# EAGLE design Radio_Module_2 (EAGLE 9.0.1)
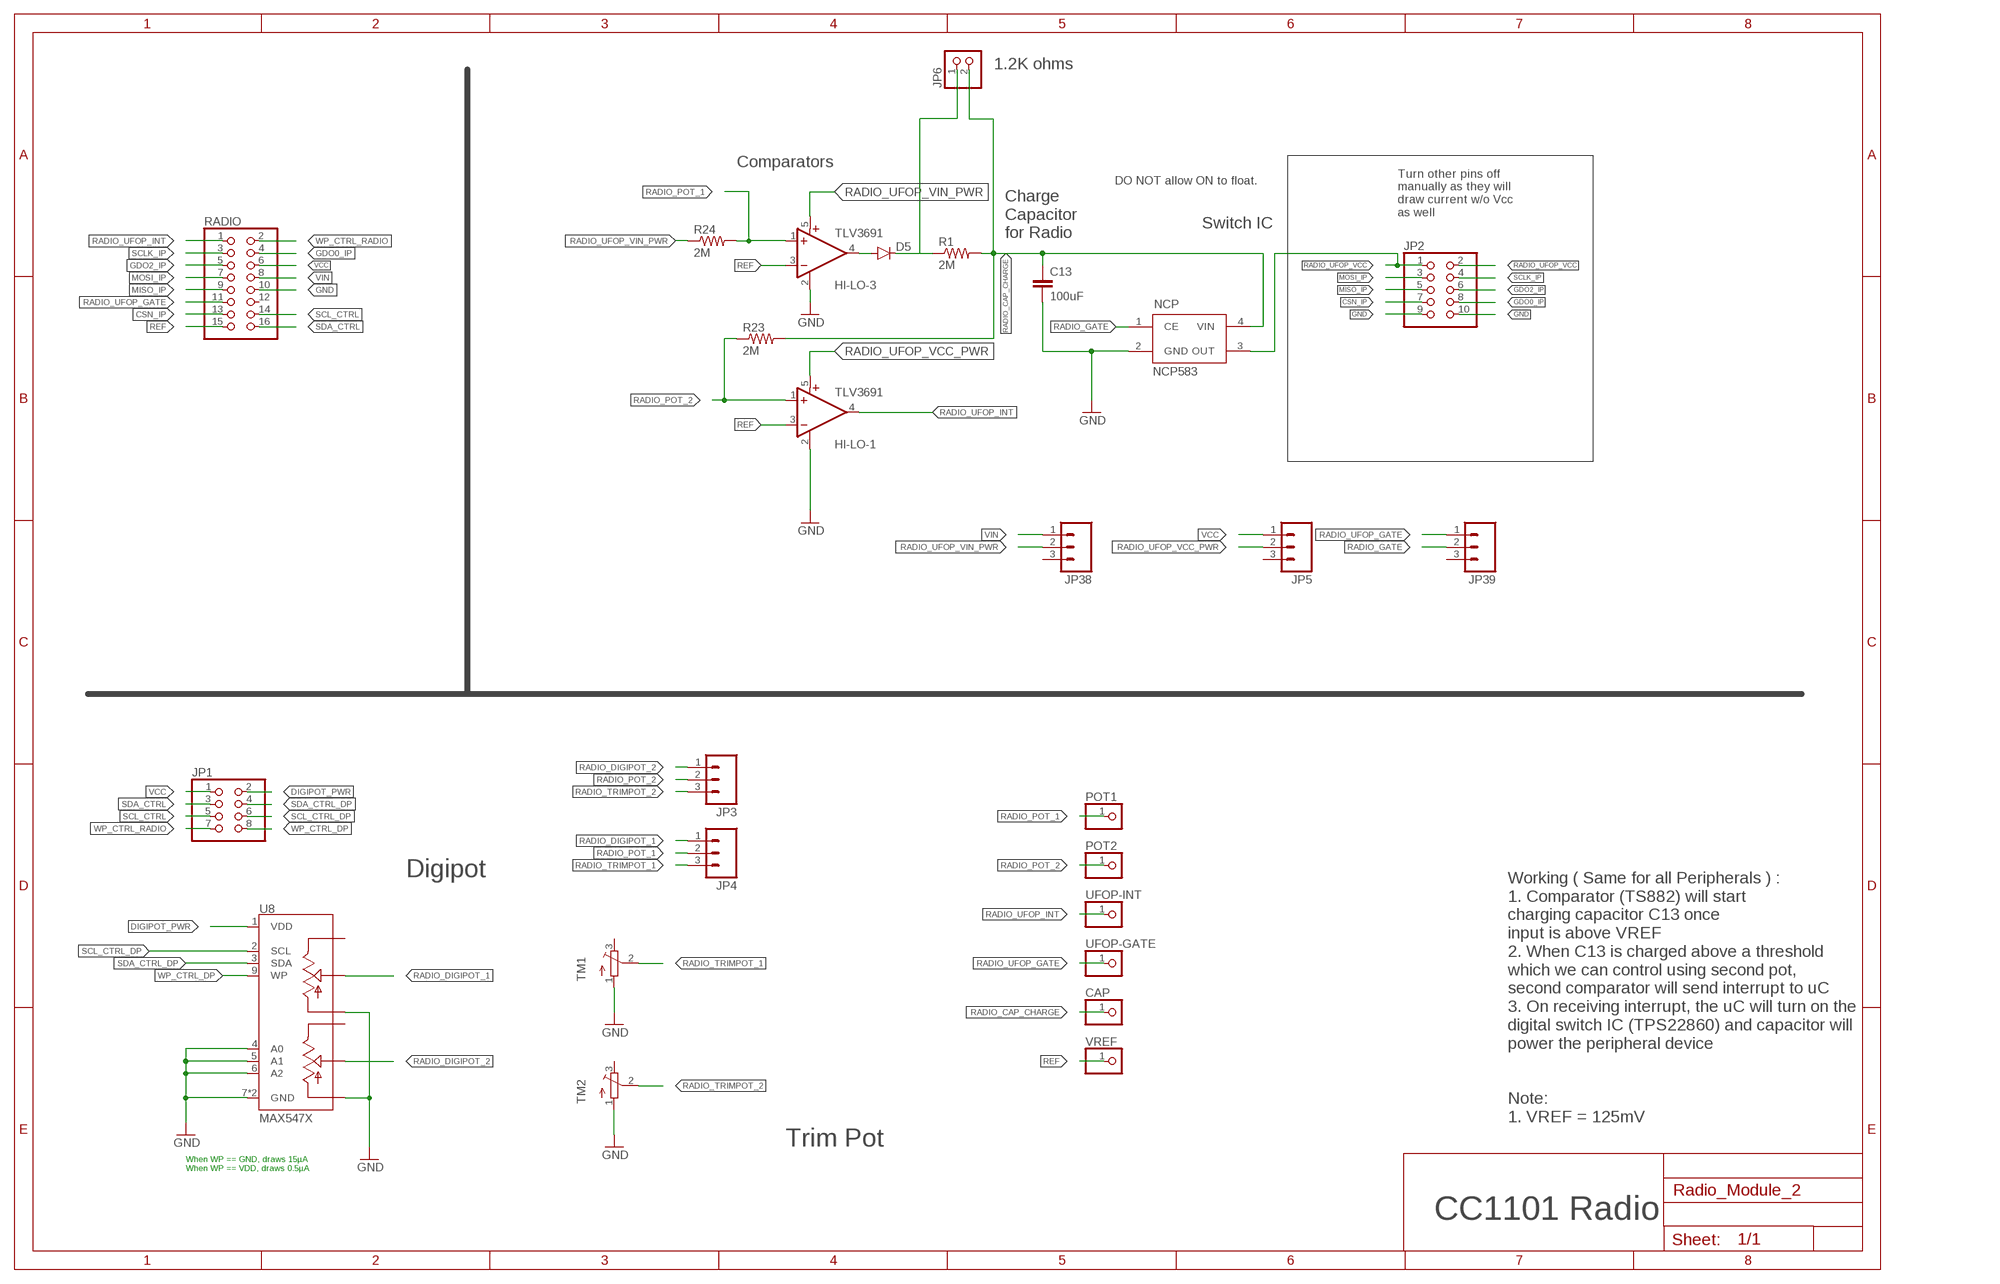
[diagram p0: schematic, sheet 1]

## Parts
C13  100uF  CAP0805  [0805]
CAP  PINHD-1X1  [1X01]
D5  DIODESOD523  [SOD523]
HI-LO-1  TLV3691  [SC70-5]
HI-LO-3  TLV3691  [SC70-5]
JP1  PINHD-2X4  [2X04]
JP2  PINHD-2X5  [2X05]
JP3  M03  [1X03-1.27MM]
JP4  M03  [1X03-1.27MM]
JP5  M03  [1X03-1.27MM]
JP6  PINHD-1X2  [1X02]
JP38  M03  [1X03-1.27MM]
JP39  M03  [1X03-1.27MM]
NCP  NCP583  [SC82-AB_1PRIMARY]
POT1  PINHD-1X1  [1X01]
POT2  PINHD-1X1  [1X01]
R1  2M  RESISTOR0805-RES  [0805]
R23  2M  RESISTOR0805-RES  [0805]
R24  2M  RESISTOR0805-RES  [0805]
RADIO  PINHD-2X8/90  [2X08/90]
TM1  TRIMPOTTC33X  [TC33X]
TM2  TRIMPOTTC33X  [TC33X]
U8  MAX547X  [QFN16]
UFOP-GATE  PINHD-1X1  [1X01]
UFOP-INT  PINHD-1X1  [1X01]
VREF  PINHD-1X1  [1X01]

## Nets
CSN_IP: JP2.7 RADIO.13
DIGIPOT_PWR: JP1.2 U8.1(VDD)
GDO0_IP: JP2.8 RADIO.4
GDO2_IP: JP2.6 RADIO.5
GND: C13.2 HI-LO-1.2(GND) HI-LO-3.2(GND) JP2.9 JP2.10 NCP.2(GND) RADIO.10 TM1.1(A) TM2.1(A) U8.4(A0) U8.5(A1) U8.6(A2) U8.7(GND) U8.10(LB) U8.13(LA) U8.TH(GND)
MISO_IP: JP2.5 RADIO.9
MOSI_IP: JP2.3 RADIO.7
N$1: D5.C JP6.1 R1.1
N$24: D5.A HI-LO-3.4(OUT)
RADIO_CAP_CHARGE: C13.1 CAP.1 JP6.2 NCP.4(VIN) R1.2 R23.2
RADIO_DIGIPOT_1: JP4.1 U8.14(WA)
RADIO_DIGIPOT_2: JP3.1 U8.11(WB)
RADIO_GATE: JP39.2 NCP.1(CE)
RADIO_POT_1: HI-LO-3.1(+IN) JP4.2 POT1.1 R24.2
RADIO_POT_2: HI-LO-1.1(+IN) JP3.2 POT2.1 R23.1
RADIO_TRIMPOT_1: JP4.3 TM1.2(S)
RADIO_TRIMPOT_2: JP3.3 TM2.2(S)
RADIO_UFOP_GATE: JP39.1 RADIO.11 UFOP-GATE.1
RADIO_UFOP_INT: HI-LO-1.4(OUT) RADIO.1 UFOP-INT.1
RADIO_UFOP_VCC: JP2.1 JP2.2 NCP.3(OUT)
RADIO_UFOP_VCC_PWR: HI-LO-1.5(V+) JP5.2
RADIO_UFOP_VIN_PWR: HI-LO-3.5(V+) JP38.2 R24.1
REF: HI-LO-1.3(-IN) HI-LO-3.3(-IN) RADIO.15 VREF.1
SCL_CTRL: JP1.5 RADIO.14
SCL_CTRL_DP: JP1.6 U8.2(SCL)
SCLK_IP: JP2.4 RADIO.3
SDA_CTRL: JP1.3 RADIO.16
SDA_CTRL_DP: JP1.4 U8.3(SDA)
VCC: JP1.1 JP5.1 RADIO.6
VIN: JP38.1 RADIO.8
WP_CTRL_DP: JP1.8 U8.9(WP)
WP_CTRL_RADIO: JP1.7 RADIO.2
Unconnected: JP5.3 JP38.3 JP39.3 RADIO.12 TM1.3(E) TM2.3(E) U8.12(HB) U8.15(HA)

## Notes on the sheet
- 1.2K ohms
- Comparators
- DO NOT allow ON to float.
- Charge 
  Capacitor 
  for Radio
- Turn other pins off 
  manually as they will
  draw current w/o Vcc
  as well
- Switch IC
- Digipot
- Working ( Same for all Peripherals ) :
  1. Comparator (TS882) will start 
  charging capacitor C13 once 
  input is above VREF
  2. When C13 is charged above a threshold
  which we can control using second pot, 
  second comparator will send interrupt to uC
  3. On receiving interrupt, the uC will turn on the
  digital switch IC (TPS22860) and capacitor will 
  power the peripheral device
- Note:
  1. VREF = 125mV
- Trim Pot
- When WP == GND, draws 15µA
  When WP == VDD, draws 0.5µA
- CC1101 Radio

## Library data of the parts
C13 = SparkFun-Capacitors:CAP: Capacitor; DIGIKEY: 490-9969-1-ND
CAP POT1 POT2 UFOP-GATE UFOP-INT VREF = adafruit:PINHD-1X1: Pin header 1x1 for 0.1" spacing
D5 = SparkFun-DiscreteSemi:DIODE: Diode
HI-LO-1 HI-LO-3 = fedpower:TLV3691: 0.9-V to 6.5-V, Nanopower Comparator Datasheets Analog Signal Chain Guide TLV3691 Manufacturer Product Page TLV3691IDPFR Specifications Standard Package 1 CategoryIntegrated Circuits (ICs) FamilyLinear - Comparators Series- Packaging Cut Tape (CT) TypeGeneral Purpose Number of Elements1 Output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
JP1 = pinhead:PINHD-2X4: PIN HEADER
JP2 = pinhead:PINHD-2X5: PIN HEADER
JP3-JP5 JP38 JP39 = SparkFun-Connectors:M03: Header 3 Standard 3-pin 0.1" header. Use with straight break away headers (SKU : PRT-00116), right angle break away headers (PRT-00553), swiss pins (PRT-00743), machine pins (PRT-00117), and female headers (PRT-00115). Molex polarized connector foot print use with SKU : PRT-08232 with associated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
JP6 = pinhead:PINHD-1X2: PIN HEADER
NCP = ncp583:NCP583: NCP583 - Ultra-Low Iq 150 mA CMOS LDO Regulator with Enable The NCP583 series of low dropout regulators are designed for portable battery powered applications which require precise output voltage accuracy and low quiescent current. These devices feature an enable function which lowers current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
R1 R23 = SparkFun-Resistors:RESISTOR: Resistor; DIGIKEY: 311-2.00MHRCT-ND
R24 = SparkFun-Resistors:RESISTOR: Resistor
RADIO = pinhead:PINHD-2X8: PIN HEADER
TM1 TM2 = adafruit:TRIMPOT: SMT trimmer potentiometer part number TC33X http://www.ladyada.net/library/eagle
U8 = max547x:MAX547X: MAXIM MAX547X: Dual, 256-Tap, Nonvolatile, I2C-Interface, Digital Potentiometers, 400nA Iq, 250µA 12ms write The MAX5477/MAX5478/MAX5479 nonvolatile, dual, linear-taper, digital potentiometers perform the function of a mechanical potentiometer, but replace the mechanics with a simple 2-wire digital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; DIGIKEY: MAX5479ETE+-ND

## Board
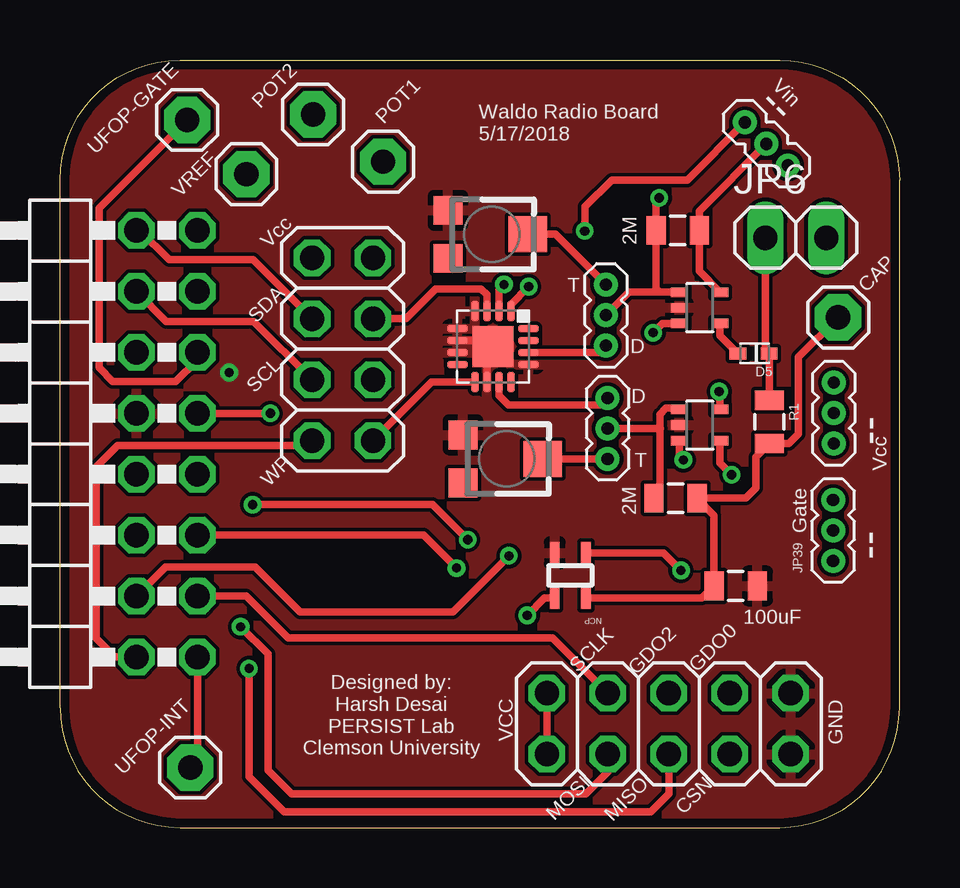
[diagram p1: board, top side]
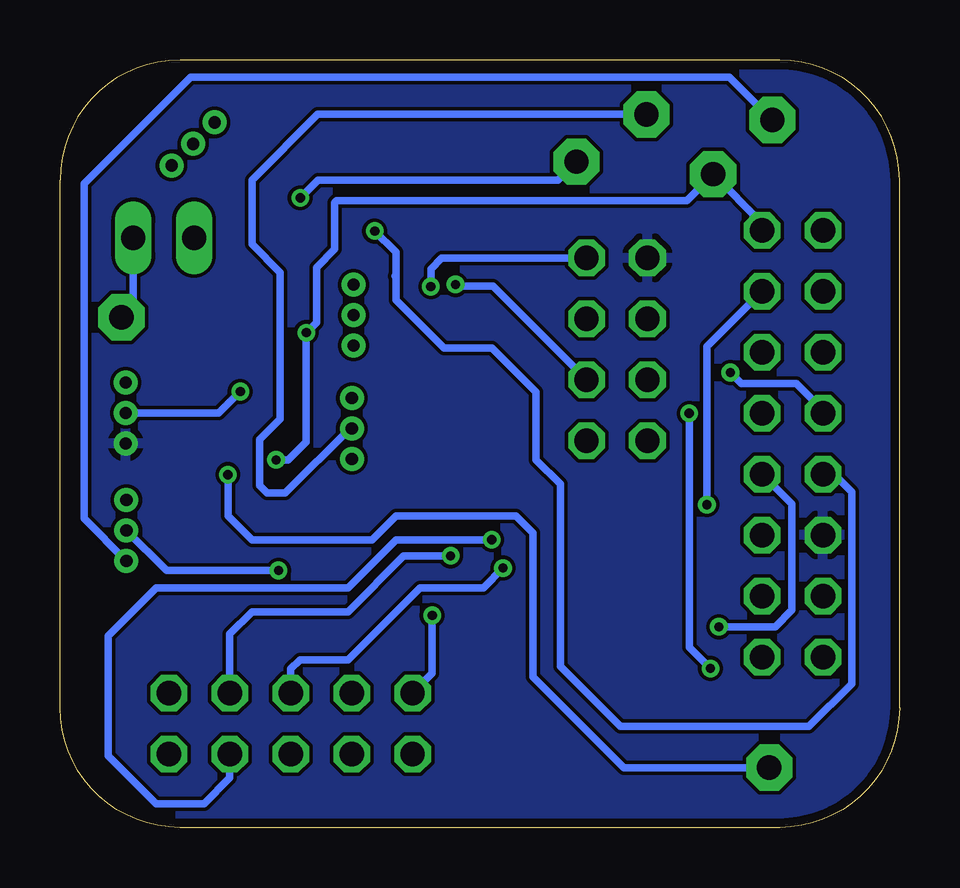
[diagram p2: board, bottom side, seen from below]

Size 35 x 32 mm. Coordinates in mm from the lower left corner, seen from the top.
Outline: 5,0 30,0 arc90 35,5 35,27 arc90 30,32 5,32 arc90 0,27 0,5 arc90 5,0
Copper layers (1*16): Top 0.0356mm / dielectric 1.5011mm / Bottom 0.0356mm
Design rules "oshpark-2layer": minimum track width 6mil, minimum drill 13mil, track to track 6mil, track to pad 6mil, pad to pad 6mil, via to via 6mil, smd to smd 6mil, copper to edge 15mil, drill to drill 6mil, minimum pad ring 7mil, minimum via ring 7mil, stop-mask expansion 2.5mil, vias tented up to drill 0mil, thermal gap 10mil

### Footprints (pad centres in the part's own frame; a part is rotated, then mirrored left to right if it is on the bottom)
0805 = smd 0.8 x 1.2: 1 -0.9,0; 2 0.9,0
1X01 = drill 1.016 pad 1.93 octagon: 1 0,0
SOD523 = smd 0.7 x 0.5: A 0.7,0; C -0.6,0
SC70-5 = smd 0.4 x 0.7: 1 -0.65,-0.85; 2 0,-0.85; 3 0.65,-0.85; 4 0.65,0.85; 5 -0.65,0.85
2X04 = drill 1.016 octagon: 1 -3.81,-1.27; 2 -3.81,1.27; 3 -1.27,-1.27; 4 -1.27,1.27; 5 1.27,-1.27; 6 1.27,1.27; 7 3.81,-1.27; 8 3.81,1.27
2X05 = drill 1.016 octagon: 1 -5.08,-1.27; 2 -5.08,1.27; 3 -2.54,-1.27; 4 -2.54,1.27; 5 0,-1.27; 6 0,1.27; 7 2.54,-1.27; 8 2.54,1.27; 9 5.08,-1.27; 10 5.08,1.27
1X03-1.27MM = drill 0.508 pad 1: 1 -1.27,0; 2 0,0; 3 1.27,0
1X02 = drill 1.016 long: 1 -1.27,0; 2 1.27,0
SC82-AB_1PRIMARY = smd 0.406 x 0.914: 1 -1.321,-0.813; 2 -0.025,-0.813; 3 -0.025,1.067; 4 -1.321,1.067
2X08/90 = drill 1.016 octagon: 1 -8.89,-6.35; 2 -8.89,-3.81; 3 -6.35,-6.35; 4 -6.35,-3.81; 5 -3.81,-6.35; 6 -3.81,-3.81; 7 -1.27,-6.35; 8 -1.27,-3.81; 9 1.27,-6.35; 10 1.27,-3.81; 11 3.81,-6.35; 12 3.81,-3.81; 13 6.35,-6.35; 14 6.35,-3.81; 15 8.89,-6.35; 16 8.89,-3.81
TC33X = smd 1.2 x 1.2: 1 -1,-1.825; 3 1,-1.825 | smd 1.5 x 1.6: 2 0,1.5
QFN16 = smd 0.85 x 0.3: 1 -1.475,0.75; 2 -1.475,0.25; 3 -1.475,-0.25; 4 -1.475,-0.75; 9 1.475,-0.75; 10 1.475,-0.25; 11 1.475,0.25; 12 1.475,0.75 | smd 0.3 x 0.85: 5 -0.75,-1.475; 6 -0.25,-1.475; 7 0.25,-1.475; 8 0.75,-1.475; 13 0.75,1.475; 14 0.25,1.475; 15 -0.25,1.475; 16 -0.75,1.475 | smd 1.7 x 1.7: TH 0,0

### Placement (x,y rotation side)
C13  28.17,10.07 0 top
CAP  32.44,21.27 0 top
D5  28.96,19.77 180 top
HI-LO-1  26.67,16.78 270 top
HI-LO-3  26.67,21.67 270 top
JP1  11.78,19.94 270 top
JP2  25.38,4.33 0 top
JP3  22.83,16.64 270 top
JP4  22.76,21.36 90 top
JP5  32.26,17.28 90 top
JP6  30.68,24.59 0 top
JP38  29.45,28.5 315 top
JP39  32.23,12.39 90 top
NCP  20.6,10.63 180 top
POT1  13.47,27.76 0 top
POT2  10.55,29.73 0 top
R1  29.57,16.92 270 top
R23  25.66,13.73 0 top
R24  25.75,24.9 180 top
RADIO  -0.62,16 90 top
TM1  18,24.73 270 top
TM2  18.63,15.37 270 top
U8  18.05,20.05 270 top
UFOP-GATE  5.3,29.5 0 top
UFOP-INT  5.43,2.5 0 top
VREF  7.77,27.24 0 top

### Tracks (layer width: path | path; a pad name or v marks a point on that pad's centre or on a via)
CSN_IP  (via drill 0.38)
  Top 0.305: v8.03,13.46 15.54,13.46 v17,12
  Bottom 0.305: v8.03,13.46 8.03,20.05 RADIO.13 | JP2.7 27.92,2.08 29,1 31,1 33,3 33,8 31,10 23,10 21,12 v17,12
DIGIPOT_PWR  (via drill 0.38)
  Top 0.305: U8.1 18.8,21.81 v19.54,22.55
  Bottom 0.305: v19.54,22.55 19.54,23.29 19.1,23.73 13.07,23.73 JP1.2
GDO0_IP  (via drill 0.38)
  Top 0.305: RADIO.4 4.4,10.86 8.14,10.86 10,9 16.39,9 v18.71,11.33
  Bottom 0.305: v18.71,11.33 20.67,11.33 23,9 27,9 27.92,8.08 JP2.8
GDO2_IP  (via drill 0.38)
  Top 0.305: RADIO.5 15.16,12.19 v16.53,10.82
  Bottom 0.305: v16.53,10.82 17.35,10 20,10 23,7 25,7 25.38,6.62 JP2.6
GND  (via drill 0.38)
  Top 0.305: U8.6 17.8,20.3 U8.TH 17.8,19.8 U8.10
  Bottom 0.305: RADIO.10 3.19,17.4 4.3,18.51 6.59,18.51 v7.05,18.97
  pour Top: -1,33 -1,-1 47,-1 47,33
MISO_IP  (via drill 0.38)
  Top 0.305: v8.77,17.27 RADIO.9 | JP2.5 25.38,1.4 24.63,0.65 9.35,0.65 7.88,2.12 v7.88,6.63
  Bottom 0.305: v8.77,17.27 8.77,7.52 v7.88,6.63
MOSI_IP  (via drill 0.38)
  Top 0.305: JP2.3 22.84,2.32 21.93,1.41 9.66,1.41 8.67,2.39 8.67,7.23 v7.53,8.37
  Bottom 0.305: RADIO.7 4.48,13.48 4.48,9.07 5.18,8.37 v7.53,8.37
N$1
  Top 0.305: R1.1 D5.C 29.41,19.92 JP6.1
N$24
  Top 0.305: HI-LO-3.4 27.52,20.51 D5.A
RADIO_CAP_CHARGE
  Top 0.305: R23.2 26.53,13.7 | 26.37,13.54 R23.2 | R23.2 28.59,13.73 29.01,14.15 29.01,15.46 R1.2 30.39,16.02 30.79,16.41 30.79,19.62 CAP.1 | R23.2 27.27,13.02 C13.1 26.77,9.57 NCP.4
  Bottom 0.305: CAP.1 31.95,21.76 JP6.2
RADIO_DIGIPOT_1
  Top 0.305: U8.14 22.47,19.8 JP4.1
RADIO_DIGIPOT_2
  Top 0.305: U8.11 18.3,18.01 18.69,17.62 22.54,17.62 JP3.1
RADIO_GATE  (via drill 0.38)
  Top 0.305: NCP.1 25.16,11.45 v25.89,10.72
  Bottom 0.305: JP39.2 30.56,10.72 v25.89,10.72
RADIO_POT_1  (via drill 0.38)
  Top 0.305: 25,22.32 HI-LO-3.1 | 25,22.32 23.72,22.32 JP4.2 | 25,22.32 24.85,22.47 R24.2 24.85,26.12 v24.98,26.25
  Bottom 0.305: v24.98,26.25 24.23,27 14.23,27 POT1.1
RADIO_POT_2
  Top 0.305: JP3.2 25,16.64 | 25,16.64 25.03,16.64 | 25,16.64 25,17.22 25.27,17.49 25.76,17.49 HI-LO-1.1 | 25,16.64 25,13.97 R23.1
  Bottom 0.305: JP3.2 22.91,16.64 25.61,13.94 26.36,13.94 26.68,14.26 26.68,16.18 25.82,17.04 25.82,23.14 27,24.32 27,27 24.27,29.73 POT2.1
RADIO_TRIMPOT_1
  Top 0.305: TM1.2 20.66,24.73 JP4.3
RADIO_TRIMPOT_2
  Top 0.305: TM2.2 JP3.3
RADIO_UFOP_GATE
  Top 0.305: RADIO.11 5.73,19.5 4.83,18.6 2.2,18.6 1.63,19.17 1.63,25.83 UFOP-GATE.1
  Bottom 0.305: UFOP-GATE.1 7.09,31.29 29.55,31.29 34,26.84 34,12.89 JP39.1
RADIO_UFOP_INT  (via drill 0.38)
  Top 0.305: RADIO.1 5.73,2.8 UFOP-INT.1 | HI-LO-1.4 27.52,15.19 v28,14.71
  Bottom 0.305: UFOP-INT.1 11.5,2.5 15.29,6.29 15.29,12.28 16,12.99 16,13 21,13 22,12 27,12 28,13 v28,14.71
RADIO_UFOP_VCC  (via drill 0.38)
  Top 0.305: JP2.2 JP2.1 | v19.48,8.84 20.21,9.57 NCP.3
  Bottom 0.305: JP2.2 19.48,6.42 v19.48,8.84
RADIO_UFOP_VCC_PWR  (via drill 0.38)
  Top 0.305: HI-LO-1.5 27.52,18.14 v27.48,18.18
  Bottom 0.305: JP5.2 28.38,17.28 v27.48,18.18
RADIO_UFOP_VIN_PWR
  Top 0.305: HI-LO-3.5 26.65,23.19 R24.1 26.65,25.7 JP38.2
REF  (via drill 0.38)
  Top 0.305: HI-LO-3.3 25.12,21.02 v24.73,20.63 | HI-LO-1.3 25.82,15.5 v25.99,15.33
  Bottom 0.305: v25.99,15.33 25.49,15.33 24.74,16.08 v24.74,20.62 v24.73,20.63 24.31,21.05 24.31,23.35 23.55,24.11 23.55,26.05 23.46,26.14 8.86,26.14 VREF.1 | 5.73,25.16 RADIO.15 5.73,25.2 VREF.1 | VREF.1
SCL_CTRL
  Top 0.305: RADIO.14 4.43,21.1 8.08,21.1 JP1.5
SCL_CTRL_DP  (via drill 0.38)
  Top 0.305: v18.51,22.64 18.3,22.43 U8.2
  Bottom 0.305: JP1.6 16.95,22.57 18.44,22.57 v18.51,22.64
SCLK_IP
  Top 0.305: RADIO.3 7.77,9.65 9.52,7.9 20.54,7.9 JP2.4
SDA_CTRL
  Top 0.305: RADIO.16 3.33,24.89 4.55,23.67 8.05,23.67 JP1.3
SDA_CTRL_DP
  Top 0.305: JP1.4 14.42,21.21 15.66,22.45 17.56,22.45 17.8,22.21 U8.3
VCC
  pour Bottom: -3,35 -3,-3 49,-3 49,35
VIN  (via drill 0.38)
  Top 0.305: v21.88,24.87 21.88,25.88 23,27 26.15,27 JP38.1
  Bottom 0.305: 21,23 21,22 19,20 17,20 15.16,18.16 15.16,15.33 14.14,14.31 14.14,6.72 11.63,4.21 3.79,4.21 2,6 2,14 2.73,14.73 RADIO.8 | 21,23 21.03,23 | 21,23 21,23.99 v21.88,24.87
WP_CTRL_DP
  Top 0.305: U8.9 15.49,18.57 JP1.8
WP_CTRL_RADIO
  Top 0.305: RADIO.2 2.29,7.11 1.51,7.89 1.51,15.04 2.4,15.93 10.31,15.93 JP1.7

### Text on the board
tPlace: -- | Vin | Waldo Radio Board / 5/17/2018 | Vcc | T | SDA | D | SCL | D | -- | T | Vcc | WP | Gate | -- | GDO0 | SCLK | GDO2 | Designed by: / Harsh Desai / PERSIST Lab / Clemson University | VCC | GND | MOSI | MISO | CSN

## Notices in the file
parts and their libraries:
SparkFun-Capacitors: Licensing: Creative Commons ShareAlike 4.0 International - https://creativecommons.org/licenses/by-sa/4.0
